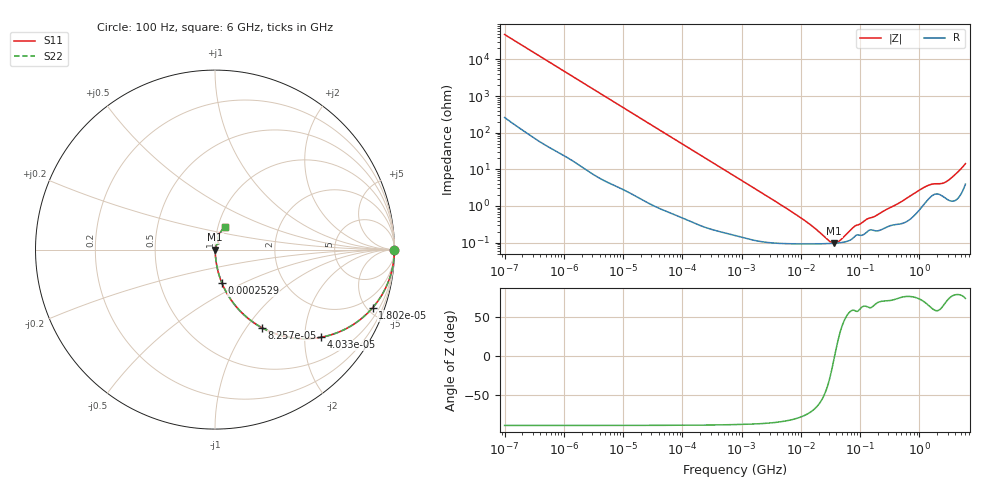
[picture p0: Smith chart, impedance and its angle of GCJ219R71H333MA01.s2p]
!Murata Part Number: GCJ219R71H333MA01
!These Parameters are Measured in Series Mode Connection
!Data Generated on Mar 13, 2026
!  o--ll--o
!Port1  Port2
!  o------o
!Operation Temp=25[degC], DC Bias Voltage=0[V]
!Freq. Start=100[Hz] Stop=6[GHz] 401[Steps]
# Hz S RI R 50
!Freq.(Hz) S11(Real) S11(Imag) S21(Real) S21(Imag) S12(Real) S12(Imag) S22(Real) S22(Imag)
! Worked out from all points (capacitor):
!   401 points, 100 Hz to 6 GHz, reference 50 ohm
!   read as one part in series: C = 33.2 nF near 109 Hz
!   lowest |Z| = 95.8 mohm at 36.42 MHz (marker M1)
!   series resonance near 37.28 MHz, so ESL is about 550 pH
!   S11 on the Smith chart (normalised r, x): 100 Hz: open; 18.02 kHz: 1.03, -5.39; 40.34 kHz: 1.02, -2.42; 82.57 kHz: 1.01, -1.18; 252.9 kHz: 1.01, -0.39; 6 GHz: 1.08, +0.27
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100  1 -0.00209  1.57e-05 0.00209  1.57e-05 0.00209  1 -0.00209
2008  0.9981 -0.0415  0.00193 0.0415  0.00193 0.0415  0.9981 -0.0415
6728  0.9804 -0.1361  0.0196 0.1361  0.0196 0.1361  0.9804 -0.1361
18016  0.8776 -0.3246  0.1224 0.3246  0.1224 0.3246  0.8776 -0.3246
26957  0.7637 -0.4215  0.2363 0.4215  0.2363 0.4215  0.7637 -0.4215
40335  0.5928 -0.4878  0.4072 0.4878  0.4072 0.4878  0.5928 -0.4878
57709  0.4176 -0.4892  0.5824 0.4892  0.5824 0.4892  0.4176 -0.4892
82567  0.2614 -0.4349  0.7386 0.4349  0.7386 0.4349  0.2614 -0.4349
135116  0.1188 -0.3184  0.8812 0.3184  0.8812 0.3184  0.1188 -0.3184
252896  0.0387 -0.1864  0.9613 0.1864  0.9613 0.1864  0.0387 -0.1864
774597  0.0056 -0.0635  0.9944 0.0635  0.9944 0.0635  0.0056 -0.0635
6075234  0.000993 -0.008  0.999 0.008  0.999 0.008  0.000993 -0.008
1.555665e7  0.000925 -0.00266  0.9991 0.00266  0.9991 0.00266  0.000925 -0.00266
2.911731e7  0.000937 -0.000673  0.9991 0.000673  0.9991 0.000673  0.000937 -0.000673
3.64232e7  0.000955 -6.27e-05  0.999 6.27e-05  0.999 6.27e-05  0.000955 -6.27e-05
4.556224e7  0.000988 0.000552  0.999 -0.000552  0.999 -0.000552  0.000988 0.000552
8.154455e7  0.00147 0.00238  0.9985 -0.00238  0.9985 -0.00238  0.00147 0.00238
3.124326e8  0.00289 0.00826  0.9971 -0.00826  0.9971 -0.00826  0.00289 0.00826
1.309207e9  0.0139 0.031  0.9861 -0.031  0.9861 -0.031  0.0139 0.031
2.802721e9  0.0174 0.0408  0.9826 -0.0408  0.9826 -0.0408  0.0174 0.0408
3.666503e9  0.0169 0.0593  0.9831 -0.0593  0.9831 -0.0593  0.0169 0.0593
6e9  0.0541 0.1247  0.9459 -0.1247  0.9459 -0.1247  0.0541 0.1247
